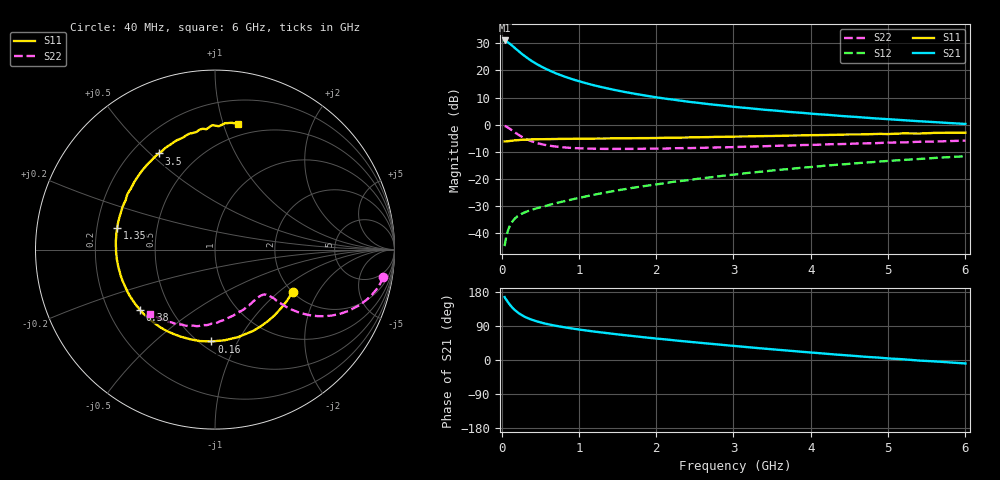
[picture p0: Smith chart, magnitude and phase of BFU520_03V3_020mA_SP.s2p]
! Filename:  P:\Prog\Test\Noise\ATS_data\Testdata_Net\03 Spar\BFU520_APG2013_37_A05_03p3V_020mA_SP_CM01_D.s2p
! Date/Time: Fri 26/Apr/2013 13:00:07
! BFU520_APG2013_37_A05_03p3V_1to20mA_SP_CM01_Bias8_R.s2p
! MDIF S-parameter v. bias file
! BFU520_APG2013_37_A05_03p3V_1to20mA_SP_CM01
! Date/time Tue Apr 23 14:11:50 2013
! VAR V_out= 3.3000
! VAR I_out= 20.0100
! VAR V_in= 0.8584
! VAR I_in= 0.2427
! Device data file deembeded for feedlines and parallel
! Original file: \03 Spar\BFU520_APG2013_37_A05_03p3V_020mA_SP_CM01_R.s2p
! Feed-files: PR047V01_250413_Feed1.s2p, PR047V01_250413_Feed2.s2p
! Parallel-file: PR047V01_250413_Par.s2p
# MHz S MA R 50
!  Freq-MHz  S11-mag  S11-arg  S21-mag  S21-arg  S12-mag  S12-arg  S22-mag  S22-arg
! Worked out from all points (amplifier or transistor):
!   98 points, 40 MHz to 6 GHz, reference 50 ohm
!   highest |S21| = 31.0 dB at 40 MHz (marker M1)
!   |S21| within 3 dB of that: start of sweep to 181.9 MHz
!   unconditionally stable (mu >= 1): 1.015 GHz to 3.142 GHz
!   at 300 MHz: K = 0.51, MSG = 28.8 dB, |S12| = -32.3 dB
!   at 1.6 GHz: K = 1.08, MAG = 16.1 dB, |S12| = -23.7 dB
!   at 6 GHz: K = 0.77, MSG = 5.9 dB, |S12| = -11.6 dB
!   S11 on the Smith chart (normalised r, x): 40 MHz: 2.01, -1.25; 160 MHz: 0.57, -0.79; 380 MHz: 0.34, -0.32; 1.35 GHz: 0.29, +0.10; 3.5 GHz: 0.31, +0.53; 6 GHz: 0.39, +1.12
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40  0.492 -28.5  35.61 166.1  0.005803 80.0  0.9498 -9.4
50  0.4921 -35.5  35.31 162.2  0.007155 78.0  0.94 -11.6
90  0.498 -59.7  32.28 150.7  0.01197 69.5  0.8746 -19.8
120  0.5042 -75.3  30.01 142.8  0.01483 64.5  0.8179 -24.7
140  0.5081 -84.2  28.41 138.3  0.01646 61.8  0.7809 -27.4
160  0.5119 -92.2  26.8 134.2  0.0179 59.4  0.7456 -29.6
200  0.5182 -105.6  23.94 127.0  0.02022 56.0  0.68 -33.0
240  0.5239 -116.4  21.46 121.2  0.02206 53.8  0.6259 -35.3
260  0.5275 -121.0  20.36 118.6  0.02288 53.0  0.6025 -36.2
320  0.5322 -132.3  17.53 112.2  0.02497 51.5  0.5447 -38.0
380  0.5362 -141.0  15.27 107.2  0.02678 51.2  0.5013 -38.9
480  0.5404 -151.8  12.53 100.6  0.02961 51.8  0.4518 -39.5
600  0.5435 -161.3  10.27 94.5  0.03287 53.5  0.4157 -39.9
800  0.5482 -172.4  7.842 86.8  0.0387 56.4  0.3837 -41.1
1050  0.5531 177.1  6.042 79.1  0.04648 59.3  0.3664 -43.6
1350  0.5578 167.6  4.729 71.3  0.05655 61.6  0.3588 -47.7
2050  0.5717 150.1  3.122 55.7  0.08128 63.3  0.3636 -60.3
3100  0.6072 127.5  2.073 35.5  0.1249 61.0  0.3913 -80.6
3500  0.6198 120.2  1.841 28.3  0.1434 58.7  0.4072 -88.2
4100  0.6454 109.2  1.56 18.2  0.1711 54.8  0.428 -100.0
5200  0.6934 91.3  1.211 1.8  0.2248 45.9  0.472 -120.8
6000  0.7137 79.8  1.034 -9.1  0.263 38.2  0.5086 -135.4
